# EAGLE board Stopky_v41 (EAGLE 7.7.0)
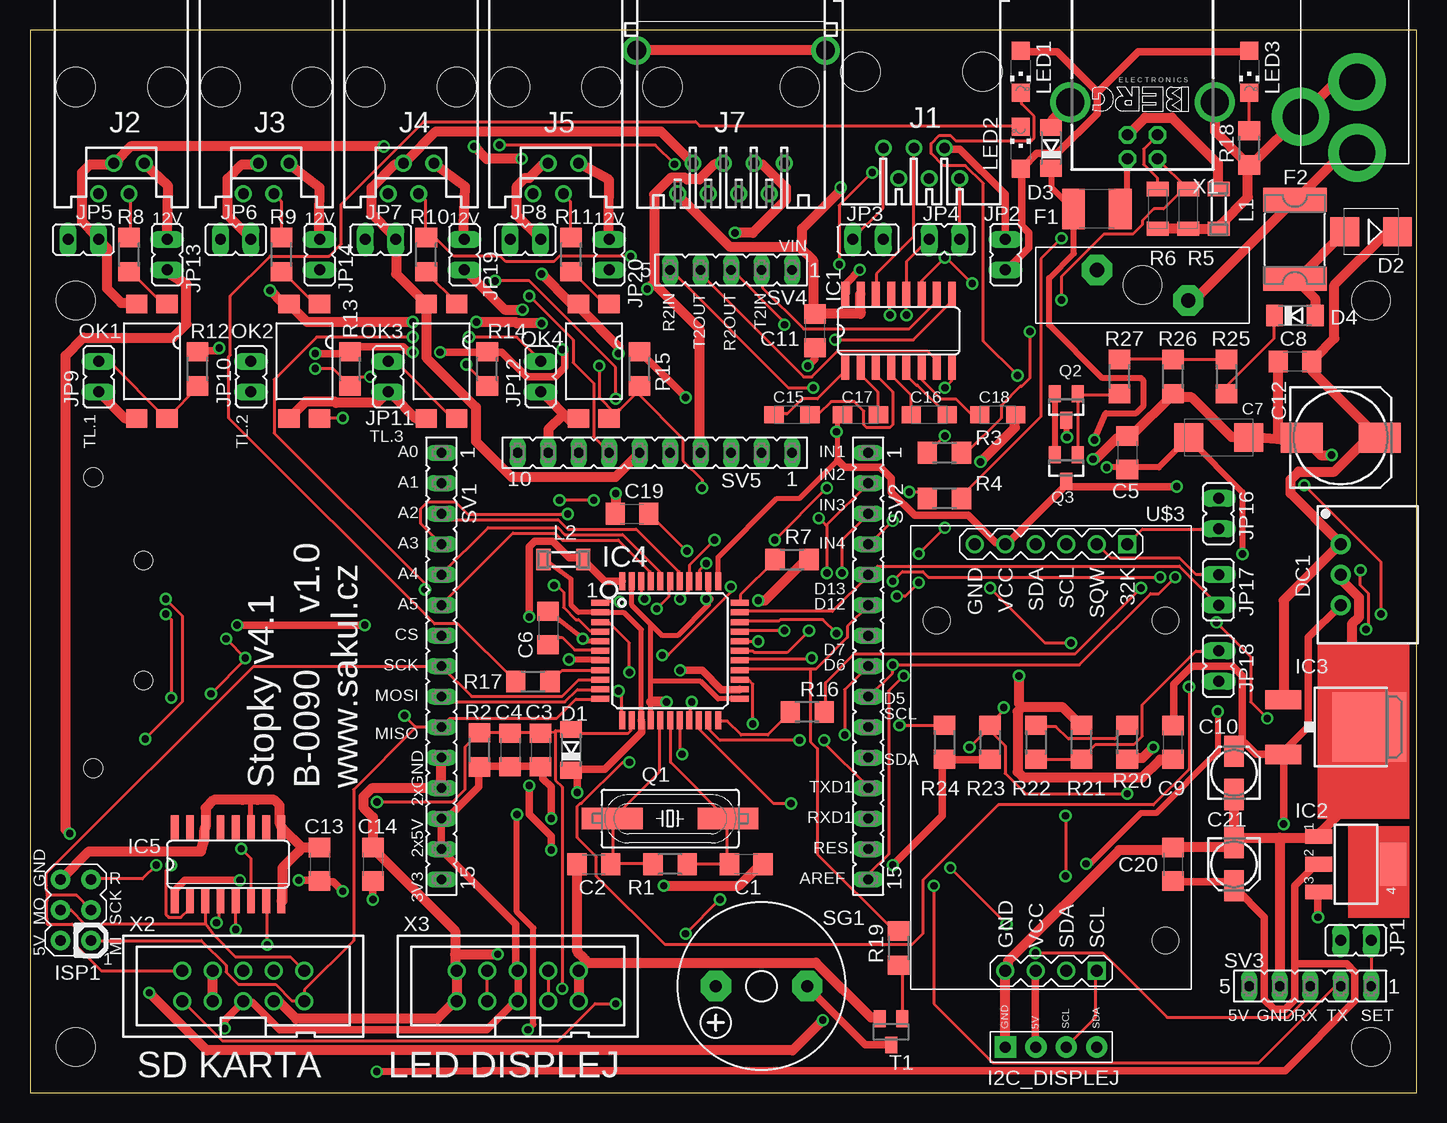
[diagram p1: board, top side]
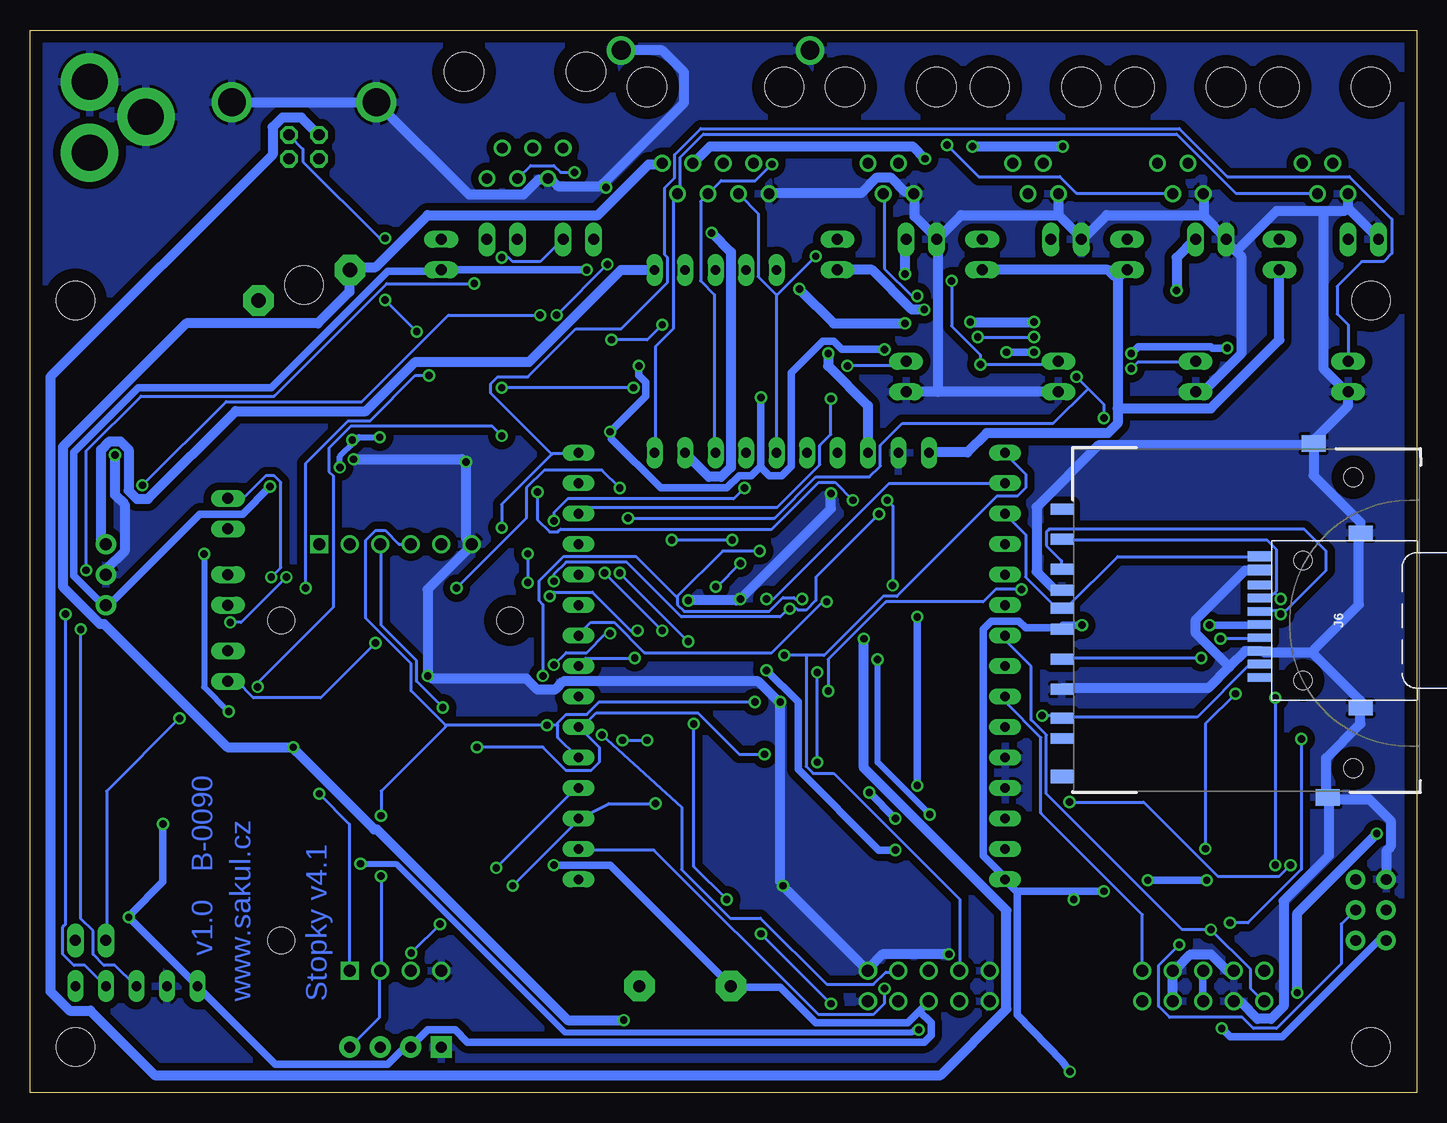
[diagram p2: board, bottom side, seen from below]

Size 115.55 x 88.57 mm. Coordinates in mm from the lower left corner, seen from the top.
Outline: 0,0 115.55,0 115.55,88.57 0,88.57 0,0
Copper layers (1*16): Top 0.035mm / dielectric 1.5mm / Bottom 0.035mm
Design rules "default": minimum track width 10mil, minimum drill 24mil, track to track 8mil, track to pad 8mil, pad to pad 8mil, via to via 8mil, smd to smd 8mil, copper to edge 40mil, drill to drill 8mil, minimum pad ring 10mil, minimum via ring 8mil, stop-mask expansion 4mil, vias tented up to drill 0mil, thermal gap 10mil
Net classes: 0 default: width 0.203 mm, drill 0.406 mm, clearance 0.203 mm; 1 12V: width 0.813 mm, drill 0.406 mm, clearance 0.203 mm; 2 5V: width 0.61 mm, drill 0.406 mm, clearance 0.203 mm; 3 GND: width 0.813 mm, drill 0.406 mm, clearance 0.203 mm; 4 3V3: width 0.61 mm, drill 0.406 mm, clearance 0.203 mm; 5 USB: width 0.508 mm, drill 0.406 mm, clearance 0.203 mm
Holes 3.2 mm at 3.81,3.81 111.76,3.81 3.81,66.04 111.76,66.04

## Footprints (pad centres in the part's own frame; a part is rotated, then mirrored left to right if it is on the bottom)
C1206 = smd 1.6 x 1.8: 1 -1.4,0; 2 1.4,0
SMC_C = smd 2.4 x 2.4: + -2.5,0; - 2.5,0
153CLV-0405 = smd 2.6 x 1.6: + 1.8,0; - -1.8,0
153CLV-0810 = smd 3.5 x 2.5: + 3.25,0; - -3.25,0
SMC_A = smd 1.6 x 1.4: + -1.5,0; - 1.5,0
SOD80C = smd 1.4 x 1.8: A 1.7,0; C -1.7,0
SMB = smd 2.4 x 2.4: A 2.2,0; C -2.2,0
SIP3 = drill 1 pad 1.676: 1 -2.54,0; 2 0,0; 3 2.54,0
L1812 = smd 1.9 x 3.4: 1 -1.95,0; 2 1.95,0
2920L = smd 2 x 5.3: 1 -3.3,0; 2 3.3,0
I2C_HEADER_FOOTPRINT = drill 0.9 pad 1.778: 5V -1.27,0; SCL 1.27,0; SDA 3.81,0 | drill 0.9 pad 1.778 square: GND -3.81,0
SO16 = smd 0.66 x 2.032: 1 -4.445,-3.073; 2 -3.175,-3.073; 3 -1.905,-3.073; 4 -0.635,-3.073; 5 0.635,-3.073; 6 1.905,-3.073; 7 3.175,-3.073; 8 4.445,-3.073; 9 4.445,3.073; 10 3.175,3.073; 11 1.905,3.073; 12 0.635,3.073; 13 -0.635,3.073; 14 -1.905,3.073; 15 -3.175,3.073; 16 -4.445,3.073
SOT223 = smd 1.219 x 2.235: 1 -2.311,-3.099; 2 0,-3.099; 3 2.311,-3.099 | smd 3.6 x 2.2: 4 0,3.099
DPACK = smd 1.6 x 3: 1 -2.28,-4.8; 3 2.28,-4.8 | smd 5.8 x 6.2: 4 0,2.38
TQFP44 = smd 1.5 x 0.5: 1 -5.8,4; 2 -5.8,3.2; 3 -5.8,2.4; 4 -5.8,1.6; 5 -5.8,0.8; 6 -5.8,0; 7 -5.8,-0.8; 8 -5.8,-1.6; 9 -5.8,-2.4; 10 -5.8,-3.2; 11 -5.8,-4; 23 5.8,-4; 24 5.8,-3.2; 25 5.8,-2.4; 26 5.8,-1.6; 27 5.8,-0.8; 28 5.8,0; 29 5.8,0.8; 30 5.8,1.6; 31 5.8,2.4; 32 5.8,3.2; 33 5.8,4 | smd 0.5 x 1.5: 12 -4,-5.8; 13 -3.2,-5.8; 14 -2.4,-5.8; 15 -1.6,-5.8; 16 -0.8,-5.8; 17 0,-5.8; 18 0.8,-5.8; 19 1.6,-5.8; 20 2.4,-5.8; 21 3.2,-5.8; 22 4,-5.8; 34 4,5.8; 35 3.2,5.8; 36 2.4,5.8; 37 1.6,5.8; 38 0.8,5.8; 39 0,5.8; 40 -0.8,5.8; 41 -1.6,5.8; 42 -2.4,5.8; 43 -3.2,5.8; 44 -4,5.8
AVRISP = drill 0.9 pad 1.626: 1 -1.27,2.54; 2 1.27,2.54; 3 -1.27,0; 4 1.27,0; 5 -1.27,-2.54; 6 1.27,-2.54
520250-3 = drill 0.889: 1 -3.175,8.89; 2 -1.905,6.35; 3 -0.635,8.89; 4 0.635,6.35; 5 1.905,8.89; 6 3.175,6.35 | hole 3.251: -5.08,0; 5.08,0
215875-3 = drill 0.889: 1 -1.905,6.35; 2 -0.635,8.89; 3 0.635,6.35; 4 1.905,8.89 | hole 3.251: -3.81,0; 3.81,0
ATTEND-112 = smd 0.85 x 2: CD 5.35,8.62; GND 4.2,8.62 | smd 0.7 x 2: CLK -1.45,8.62; CMD 0.75,8.62; DAT0 -3.65,8.62; DAT1 -4.75,8.62; DAT2 2.95,8.62; DAT3 1.85,8.62; VDD -0.35,8.62; VSS -2.55,8.62 | smd 1.2 x 2: S1 -7.3,0.22; S2 7.3,0.22 | hole 1.5: -5,5.02; 5,5.02
555153-1 = drill 0.889: 1 -4.445,6.35; 2 -3.175,8.89; 3 -1.905,6.35; 4 -0.635,8.89; 5 0.635,6.35; 6 1.905,8.89; 7 3.175,6.35; 8 4.445,8.89 | drill 1.575 pad 2.184: G1 -7.874,-3.048; G2 7.874,-3.048 | hole 3.251: -5.715,0; 5.715,0
JP1 = drill 0.914 long: 1 0,-1.27; 2 0,1.27
SM-1206 = smd 1.2 x 1.8: 1 -1.65,0; 2 1.65,0
CHIPLED_1206 = smd 1.5 x 1.5: A 0,-1.75; C 0,1.75
SMD4-7 = smd 1.78 x 1.55: 1 -1.27,-4.77; 2 1.27,-4.77; 3 1.27,4.77; 4 -1.27,4.77
SM49 = smd 5.08 x 1.778: 1 -4.826,0; 2 4.826,0
SOT23 = smd 1 x 1.4: 1 -0.95,-1.1; 2 0.95,-1.1; 3 0,1.1
R1206 = smd 1.6 x 1.803: 1 -1.422,0; 2 1.422,0
CT/CN1206 = smd 1.2 x 1.8: 1 -1.65,0; 2 1.65,0
F/CM12P = drill 1.016 pad 2.54 octagon: + 3.81,0; - -3.81,0
FE15 = drill 0.813 long: 1 -17.78,0; 2 -15.24,0; 3 -12.7,0; 4 -10.16,0; 5 -7.62,0; 6 -5.08,0; 7 -2.54,0; 8 0,0; 9 2.54,0; 10 5.08,0; 11 7.62,0; 12 10.16,0; 13 12.7,0; 14 15.24,0; 15 17.78,0
FE05-1 = drill 0.813 long: 1 -5.08,0; 2 -2.54,0; 3 0,0; 4 2.54,0; 5 5.08,0
FE10 = drill 0.813 long: 1 -11.43,0; 2 -8.89,0; 3 -6.35,0; 4 -3.81,0; 5 -1.27,0; 6 1.27,0; 7 3.81,0; 8 6.35,0; 9 8.89,0; 10 11.43,0
SDCARD-SOCKET = smd 1.8 x 0.9: 1 -1,6.77; 2 -1,4.27; 3 -1,2.52; 4 -1,-0.73; 5 -1,-3.23; 6 -1,-5.73; 7 -1,-8.15; 8 -1,-9.85; 9 -1,9.27; CD -1,1.02 | smd 2 x 1.4: SH@1 20,14.75; SH@2 21.15,-14.75 | smd 1.8 x 1.1: WP -1,-13 | hole 1.55: 23.3,11.94; 23.3,-12.32
SL-1538 = drill 1.2 pad 2.54 octagon: P$1 3.81,-1.27; P$2 -3.81,1.27 | hole 3.2: 0,0
PJ-102A = drill 3 pad 4.8: RING 0.1,-3.39; RING_SW -4.6,-6.29; TIP 0.1,-9.29
RTC-DS3231-AT24C32 = drill 1 square: J1.1 -17.78,6.35; J2.1 17.78,3.81 | drill 1: J1.2 -17.78,3.81; J1.3 -17.78,1.27; J1.4 -17.78,-1.27; J1.5 -17.78,-3.81; J1.6 -17.78,-6.35; J2.2 17.78,1.27; J2.3 17.78,-1.27; J2.4 17.78,-3.81 | hole 2.2: -11.43,-9.525; -11.43,9.525; 15.24,9.525
PN61729-S = drill 0.95 octagon: 1 1.25,4.71; 2 -1.25,4.71; 3 -1.25,2.71; 4 1.25,2.71 | drill 2.3 pad 2.9: S1 -6.02,0; S2 6.02,0
PAK100/2500-10 = drill 1 pad 1.422: 1 -5.08,-1.27; 2 -5.08,1.27; 3 -2.54,-1.27; 4 -2.54,1.27; 5 0,-1.27; 6 0,1.27; 7 2.54,-1.27; 8 2.54,1.27; 9 5.08,-1.27; 10 5.08,1.27

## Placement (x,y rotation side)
C1  22pF  [C1206]  59.69,19.05 180 top
C2  22pF  [C1206]  46.99,19.05 0 top
C3  100nF  [C1206]  42.55,28.57 270 top
C4  100nF  [C1206]  40.01,28.57 270 top
C5  100nF  [C1206]  91.44,53.34 270 top
C6  1uF  [C1206]  43.18,38.73 270 top
C7  10uF  [SMC_C]  99.06,54.61 0 top
C8  100nF  [C1206]  105.41,60.96 0 top
C9  100nF  [C1206]  95.25,29.21 90 top
C10  10uF/10V  [153CLV-0405]  100.33,26.67 90 top
C11  100nF  [C1206]  65.41,63.5 270 top
C12  220uF/35V  [153CLV-0810]  109.22,54.61 0 top
C13  100nF  [C1206]  24.13,19.05 270 top
C14  100nF  [C1206]  28.57,19.05 270 top
C15  1uF  [SMC_A]  63.5,56.52 0 top
C16  1uF  [SMC_A]  74.93,56.52 0 top
C17  1uF  [SMC_A]  69.22,56.52 180 top
C18  1uF  [SMC_A]  80.64,56.52 180 top
C19  100nF  [C1206]  50.16,48.26 0 top
C20  100nF  [C1206]  95.25,19.05 270 top
C21  10uF/10V  [153CLV-0405]  100.33,19.05 270 top
D1  1N4148  [SOD80C]  45.09,28.57 90 top
D2  STPS340U (TME)  [SMB]  111.76,71.75 180 top
D3  5V6  [SOD80C]  85.09,78.74 90 top
D4  1N4148  [SOD80C]  105.41,64.77 0 top
DC1  R-785.0-0.5  [SIP3]  109.22,43.18 270 top
F1  MF-MSMF050-2 500mA  [L1812]  88.9,73.66 180 top
F2  SL125-33 (TME)  [2920L]  105.41,71.12 90 top
I2C_DISPLEJ  I2C Display  [I2C_HEADER_FOOTPRINT]  85.09,3.81 0 top
IC1  MAX232  [SO16]  72.39,63.5 0 top
IC2  LM1117 3V3  [SOT223]  110.49,19.05 270 top
IC3  78M05 DPAK (LF50CDT)  [DPACK]  109.22,30.48 270 top
IC4  ATMEGA32U4-AU  [TQFP44]  53.34,36.83 0 top
IC5  4050D  [SO16]  16.51,19.05 0 top
ISP1  AVRISP-6  [AVRISP]  3.81,15.24 180 top
J1  [520250-3]  74.3,85.09 180 top
J2  [215875-3]  7.62,83.82 180 top
J3  [215875-3]  19.68,83.82 180 top
J4  [215875-3]  31.75,83.82 180 top
J5  [215875-3]  43.81,83.82 180 top
J6  ATTEND-MICROSD-112  [ATTEND-112]  4.45,39.37 90 bottom
J7  [555153-1]  58.42,83.82 180 top
JP1  [JP1]  110.49,12.7 270 top
JP2  [JP1]  81.28,69.85 0 top
JP3  [JP1]  69.85,71.12 90 top
JP4  [JP1]  76.2,71.12 270 top
JP5  [JP1]  4.45,71.12 90 top
JP6  [JP1]  17.14,71.12 90 top
JP7  [JP1]  29.21,71.12 90 top
JP8  [JP1]  41.27,71.12 90 top
JP9  [JP1]  5.71,59.69 0 top
JP10  [JP1]  18.41,59.69 0 top
JP11  [JP1]  29.84,59.69 0 top
JP12  [JP1]  42.55,59.69 0 top
JP13  [JP1]  11.43,69.85 0 top
JP14  [JP1]  24.13,69.85 0 top
JP16  [JP1]  99.06,48.26 180 top
JP17  [JP1]  99.06,41.91 180 top
JP18  [JP1]  99.06,35.56 180 top
JP19  [JP1]  36.2,69.85 0 top
JP20  [JP1]  48.26,69.85 0 top
L1  MH2029-300Y (1206)  [SM-1206]  99.06,73.66 90 top
L2  MH2029-300Y (1206)  [SM-1206]  44.45,44.45 180 top
LED1  [CHIPLED_1206]  82.55,85.09 180 top
LED2  [CHIPLED_1206]  82.55,78.74 0 top
LED3  [CHIPLED_1206]  101.6,85.09 180 top
OK1  SFH618A  [SMD4-7]  10.16,60.96 180 top
OK2  SFH618A  [SMD4-7]  22.86,60.96 180 top
OK3  SFH618A  [SMD4-7]  34.29,60.96 180 top
OK4  SFH618A  [SMD4-7]  46.99,60.96 180 top
Q1  16MHz  [SM49]  53.34,22.86 0 top
Q2  IRLML6402TRPBF  [SOT23]  86.36,57.15 180 top
Q3  IRLML6402TRPBF  [SOT23]  86.36,52.07 180 top
R1  1M  [R1206]  53.34,19.05 0 top
R2  10K  [R1206]  37.47,28.57 270 top
R3  22R  [R1206]  76.2,53.34 0 top
R4  22R  [R1206]  76.2,49.53 0 top
R5  B72520T040M62 (Varistor)  [CT/CN1206]  96.52,73.66 270 top
R6  B72520T040M62 (Varistor)  [CT/CN1206]  93.98,73.66 270 top
R7  10K  [R1206]  63.5,44.45 180 top
R8  3K9  [R1206]  8.26,69.85 270 top
R9  3K9  [R1206]  20.95,69.85 270 top
R10  3K9  [R1206]  33.02,69.85 270 top
R11  3K9  [R1206]  45.09,69.85 270 top
R12  10K  [R1206]  13.97,60.33 270 top
R13  10K  [R1206]  26.67,60.33 270 top
R14  10K  [R1206]  38.1,60.33 270 top
R15  10K  [R1206]  50.8,60.33 270 top
R16  1K  [R1206]  64.77,31.75 0 top
R17  1K  [R1206]  41.91,34.29 180 top
R18  1K  [R1206]  101.6,78.74 90 top
R19  10K  [R1206]  72.39,12.06 90 top
R20  10K  [R1206]  91.44,29.21 270 top
R21  2K2  [R1206]  87.63,29.21 270 top
R22  1K  [R1206]  83.82,29.21 90 top
R23  10K  [R1206]  80.01,29.21 90 top
R24  10K  [R1206]  76.2,29.21 90 top
R25  10K  [R1206]  99.69,59.69 90 top
R26  2K2  [R1206]  95.25,59.69 270 top
R27  10R  [R1206]  90.81,59.69 270 top
SG1  F/CM12P  [F/CM12P]  60.96,8.89 180 top
SV1  [FE15]  34.29,35.56 270 top
SV2  [FE15]  69.85,35.56 270 top
SV3  HC11/12  [FE05-1]  106.68,8.89 180 top
SV4  [FE05-1]  58.42,68.58 180 top
SV5  [FE10]  52.07,53.34 180 top
T1  BC846  [SOT23]  71.75,5.08 180 top
U1  [SDCARD-SOCKET]  28.57,39.37 0 bottom
U$1  ASL-1538 2A  [SL-1538]  92.71,67.31 180 top
U$2  2.1MMJACKTHM  [PJ-102A]  110.49,87.63 0 top
U$3  RTC-DS3231-AT24C32  [RTC-DS3231-AT24C32]  85.09,27.94 270 top
X1  PN61729-S  [PN61729-S]  92.71,82.55 180 top
X2  2510-  [PAK100/2500-10]  17.78,8.89 0 top
X3  2510-  [PAK100/2500-10]  40.64,8.89 0 top

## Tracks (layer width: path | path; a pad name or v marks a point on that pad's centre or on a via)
+3V3  (via drill 0.61)
  Top 0.61: C20.2 95.33,17.6 99.9,17.6 100.24,17.26 C21.+ 100.47,17.03 102.87,14.63 102.87,7.77 103.67,6.97 104.58,6.97 105.39,7.77 105.39,10.74 | 105.39,10.74 105.39,17.26 107.1,18.97 107.33,18.97 IC2.2 | v26.06,16.8 25.26,17.6 24.23,17.6 C13.2 23.89,17.72 v22.4,17.72 | v28.57,16.12 C14.2 | v27.89,38.98 v17.26,38.98 | v17.49,17.72 12.92,17.72 12.12,16.92 12.12,16 IC5.1 | 105.39,10.74 109.73,10.74 110.41,10.06 110.41,7.66 104.58,1.83 37.72,1.83 v28.89,1.76
  Bottom 0.61: 33.26,16.8 33.38,16.8 34.29,17.72 SV1.15 34.4,18.06 36.12,19.77 36.12,38.63 35.43,39.32 33.15,39.32 32.58,38.75 29.6,38.75 U1.4 29.49,38.98 v27.89,38.98 | 33.26,16.8 28.57,16.8 | 28.57,16.8 v26.06,16.8 | 28.57,16.8 v28.57,16.12 | v17.26,38.98 13.14,38.98 J6.VDD | v22.4,17.72 v17.49,17.72 | v28.89,1.76 29.53,2.63 33.26,6.51 33.26,16.8
+5V  (via drill 0.61)
  Top 0.406: IC4.14 50.94,38.59 49.53,40.01 47.56,40.01 IC4.2 45.7,40.03 45.09,40.64 45.09,42.8 L2.2 | IC4.34 57.34,44.64 62.23,49.53 64.14,49.53 67.31,52.7 67.31,55.09 67.31,56.11 C17.-
  Top 0.61: R23.1 80.01,27.77 76.24,27.77 R24.1 76.01,27.55 76.01,23.09 v71.89,18.97 | v16.23,5.37 16.23,6.06 17.72,7.54 X2.5 18.06,7.54 18.52,7.54 20.8,5.26 38.06,5.26 40.35,7.54 X3.5 40.69,7.66 40.69,10.06 X3.6 40.46,10.4 40.46,14.06 34.4,20.12 SV1.14 SV1.13 34.52,22.97 34.86,22.97 37.38,25.49 37.38,26.86 R2.2 37.49,27.2 40.01,27.2 C4.2 40.23,27.2 42.52,27.2 C3.2 42.75,26.98 42.75,26.18 43.43,25.49 v43.43,22.86 | IC4.14 50.98,30.86 50.98,30.06 47.89,26.98 45.15,26.98 D1.C 45.61,26.75 v45.61,25.03 | v15.77,62.06 15.54,61.84 14.06,61.84 R12.1 | v23.77,61.61 26.52,61.61 26.63,61.72 R13.1 26.98,61.84 27.32,62.18 31.09,62.18 31.55,61.72 v31.89,61.72 | v34.18,61.72 38.06,61.72 R14.1 38.41,61.72 39.32,61.72 41.38,59.66 43.78,59.66 44.58,60.47 44.58,61.72 v44.35,61.95 | v64.81,60.58 65.38,61.15 65.38,62.06 C11.2 | v67.21,55.09 67.31,55.09 | v54.63,57.95 50.86,61.72 R15.1 | 67.31,52.7 67.89,52.12 70.87,52.12 71.78,51.21 71.78,50.06 73.72,48.12 78.18,48.12 80.47,45.83 81.04,45.83 U$3.J1.5 81.38,45.72 86.3,50.63 86.3,50.86 Q3.3 86.53,50.52 v95.56,50.52 | JP2.1 81.38,68.58 83.21,70.41 83.21,71.67 82.64,72.24 82.64,76.92 LED2.A 82.75,77.15 83.9,78.3 85.61,78.3 88.92,81.61 88.92,83.44 | 88.92,83.44 85.61,86.75 82.64,86.75 LED1.A | LED3.A 101.5,86.75 92.35,86.75 89.15,83.55 88.92,83.44 | v69.15,68.58 68.01,67.44 68.01,66.64 IC1.16 | 101.04,29.26 101.04,34.75 100.24,35.55 96.81,35.55 95.33,34.06 95.33,30.63 C9.2 | 101.04,29.26 100.36,28.57 C10.+ | IC3.3 104.36,28.23 102.18,28.23 101.27,29.15 101.04,29.26 | DC1.3 106.53,37.95 106.53,30.52 104.47,28.46 IC3.3
  Top 0.61: U$3.J2.3 83.78,10.06 83.78,3.89 I2C_DISPLEJ.5V | v107.33,14.63 107.33,16.69 IC2.3 | v104.47,22.4 104.47,27.89 IC3.3
  Bottom 0.61: v71.89,18.97 67.21,18.97 57.15,8.91 SG1.+ 56.92,8.8 53.03,8.8 50.06,5.83 42.41,5.83 41.43,6.8 | X2.5 17.83,7.66 17.83,10.06 X2.6 | v16.23,5.37 15.54,4.69 11.2,4.69 3.2,12.69 2.63,12.69 ISP1.2 | v43.43,22.86 v45.61,25.03 | 41.43,6.8 40.69,7.54 X3.5 | v15.77,62.06 17.03,62.06 17.14,62.18 23.2,62.18 v23.77,61.61 | v31.89,61.72 v34.18,61.72 | v64.81,60.58 64.81,59.78 64.24,59.21 64.24,58.06 v67.21,55.09 67.09,54.86 67.09,54.52 62.98,50.41 57.49,50.41 56.46,51.44 55.44,51.44 54.63,52.23 | 54.63,52.23 v54.63,57.95 | v44.35,61.95 47.89,61.95 48.58,62.64 49.49,62.64 52.12,60.01 52.12,52.23 52.92,51.44 53.95,51.44 54.52,52.01 54.63,52.23 | v69.15,68.58 JP2.1 81.5,68.47 85.72,68.47 95.44,58.75 106.53,58.75 111.9,53.38 111.9,43.09 109.5,40.69 109.27,40.69 DC1.3 108.93,40.69 101.38,48.23 97.84,48.23 v95.56,50.52 | v104.47,22.4 104.47,17.6 107.21,14.86 v107.33,14.63 101.61,8.91 SV3.5 101.38,8.69 95.1,2.4 85.72,2.4 84.35,3.77 83.9,3.77 I2C_DISPLEJ.5V 83.67,4 82.41,5.26 80.12,5.26 79.1,4.23 41.03,4.23 40.46,4.8 40.46,5.83 41.43,6.8
+12V  (via drill 0.61)
  Top 0.813: v41.03,65.27 39.55,65.27 36.23,68.58 JP19.1 | v93.61,28.8 92.7,27.89 91.44,27.89 R20.2 | JP13.1 11.43,68.35 13.03,67.39 13.03,64.06 11.9,62.93 4.46,62.93 2.97,61.44 2.97,21.95 v3.31,21.6 | v9.94,8.34 14.74,3.54 63.55,3.54 v66.06,6.06
  Bottom 0.813: 24.92,57.04 24.92,67.89 24.23,68.58 JP14.1 25.26,68.12 25.72,68.58 JP19.1 | 24.92,57.04 24.92,55.78 25.72,54.98 35.84,54.98 37.44,53.38 40.58,53.38 SV5.10 | JP13.1 11.43,62.75 17.14,57.04 24.92,57.04 | JP20.1 45.38,68.58 42.06,65.27 v41.03,65.27 | J7.1 62.87,77.38 64.01,77.38 68.24,73.15 82.41,73.15 86.75,68.81 88.58,68.81 U$1.P$1 88.92,68.58 88.92,66.75 91.55,64.12 102.53,64.12 112.81,53.84 112.81,42.18 109.73,39.09 109.39,39.09 99.1,28.8 v93.61,28.8 93.38,28.46 86.87,21.95 86.64,21.95 70.75,6.06 v66.06,6.06 | v3.31,21.6 9.94,14.97 v9.94,8.34
A0  (via drill 0.61)
  Top 0.254: X3.3 38.06,7.66 38.06,10.06 X3.4 | v56.35,44.12 55.78,43.55 55.78,42.63 IC4.36 | v58.41,42.18 58.41,41.72 53.15,36.46 v52.69,36.46
  Bottom 0.254: v56.35,44.12 58.29,42.18 v58.41,42.18 | 50.86,36.46 49.38,36.46 44.46,41.38 43.32,41.38 34.98,49.72 33.26,49.72 32.58,50.41 32.58,51.55 34.29,53.26 SV1.1 | 50.86,36.46 v52.69,36.46 | 50.86,36.46 50.86,27.2 50.29,26.63 48.58,26.63 38.06,16.12 38.06,10.17 X3.4
A1  (via drill 0.61)
  Top 0.254: v54.18,41.15 54.86,41.83 54.86,42.52 IC4.37 54.98,42.75 54.98,44.01 v57.04,46.06 | v86.75,37.49 84.58,37.49 v80.01,42.06 | v62.06,46.06 v66.41,50.41
  Bottom 0.254: v54.18,41.15 53.61,41.15 44.01,50.75 34.29,50.75 SV1.2 | JP18.2 98.3,34.29 96.93,32.92 91.33,32.92 v86.75,37.49 | v80.01,42.06 74.18,47.89 74.18,50.41 72.69,51.89 67.89,51.89 v66.41,50.41 | v57.04,46.06 v62.06,46.06
A2
  Top 0.254: IC4.38 54.06,42.63 54.06,43.43 50.52,46.98 44.81,46.98 44.01,47.78 34.75,47.78 34.29,48.23 SV1.3
  Bottom 0.254: SV1.3 34.29,48.23 32.58,46.52 32.58,42.98 30.06,40.46 29.6,40.46 U1.CD 29.49,40.46 29.15,40.46 24.92,44.69 13.14,44.69 J6.CD
A3  (via drill 0.61)
  Top 0.254: v52.23,40.35 53.26,41.38 53.26,42.52 IC4.39 | v44.81,48.23 36.46,48.23 35.43,49.26 33.15,49.26 32.58,48.69 32.58,47.43 SV1.4 | v103.1,31.2 101.73,32.58 101.73,36.35 v98.87,39.2 | v94.18,42.98 74.87,42.98 74.41,43.43 72.69,43.43 v71.89,42.63
  Bottom 0.254: v44.81,48.23 50.06,42.98 50.06,41.03 50.86,40.23 51.55,40.23 51.66,40.35 v52.23,40.35 52.35,40.35 53.03,39.66 61.27,39.66 65.84,44.23 70.87,44.23 71.89,43.2 v71.89,42.63 | v103.1,31.2 109.16,25.15 109.16,12.8 JP1.1 | v98.87,39.2 97.95,39.2 v94.18,42.98
A4
  Top 0.254: IC4.40 52.46,42.63 52.46,43.43 49.38,46.52 44.58,46.52 44.01,47.09 38.18,47.09 34.29,43.2 SV1.5
A5
  Top 0.254: IC4.41 51.66,42.63 51.66,43.43 49.03,46.06 44.35,46.06 43.78,46.63 40.23,46.63 34.29,40.69 SV1.6
AREF  (via drill 0.61)
  Top 0.254: v51.21,41.15 50.98,41.38 50.98,42.52 IC4.42 | v54.75,45.15 51.66,48.23 C19.2 | v72.81,34.75 71.55,33.49 71.55,19.89 69.95,18.29 69.95,17.83 SV2.15
  Bottom 0.254: v51.21,41.15 51.78,41.15 51.89,41.26 52.81,41.26 53.95,40.12 61.04,40.12 61.61,40.69 61.61,41.38 | 61.61,41.38 57.84,45.15 v54.75,45.15 | v72.81,34.75 72.81,40.69 73.15,41.03 73.15,42.63 71.09,44.69 65.04,44.69 61.72,41.38 61.61,41.38
CS  (via drill 0.61)
  Top 0.254: v60.24,30.75 60.24,34.06 59.89,34.4 59.21,34.4 IC4.25 | v54.63,13.26 v57.49,16.12 | v48.81,7.43 47.09,7.43 44.01,4.34 16,4.34 12.8,7.54 X2.1 | v17.14,13.6 IC5.5
  Bottom 0.254: v60.24,30.75 60.24,18.86 v57.49,16.12 | v48.81,7.43 v54.63,13.26 | X2.1 12.8,7.66 13.83,8.69 13.83,10.29 v17.14,13.6 19.55,13.6 30.86,24.92 30.86,29.83 32.12,31.09 32.12,35.55 34.29,37.72 SV1.7
D5  (via drill 0.61)
  Top 0.254: v67.21,38.29 66.06,39.43 62.52,39.43 62.41,39.32 59.21,39.32 IC4.31 | SV2.9 69.95,33.03 71.89,34.98 v71.89,35.66 87.44,35.66 93.38,41.6 94.07,41.6 v95.44,42.98
  Bottom 0.254: v67.21,38.29 67.55,38.29 69.15,36.69 70.87,36.69 v71.89,35.66 | v95.44,42.98 94.64,43.78 94.64,50.86 95.21,51.44 95.9,51.44 97.73,49.61 98.98,49.61 JP16.1
D6  (via drill 0.61)
  Top 0.254: X3.7 43.2,7.66 43.2,10.06 X3.8 | v65.15,36.23 65.04,36.12 59.21,36.12 IC4.27 | v67.89,29.83 67.89,33.6 SV2.8
  Bottom 0.254: v65.15,36.23 69.27,36.23 69.84,35.66 SV2.8 | v67.89,29.83 61.24,23.81 61.24,18.61 57.2,14.57 54.69,14.57 49.15,9.03 45.26,9.03 44.23,10.06 43.2,10.06 X3.8
D7  (via drill 0.61)
  Top 0.254: v49.15,40.92 47.55,40.92 IC4.1
  Bottom 0.254: v49.15,40.92 49.49,40.92 53.72,36.69 64.35,36.69 66.86,39.2 68.81,39.2 69.84,38.18 SV2.7
D12
  Top 0.254: 65.04,35.32 65.49,35.32 68.12,37.95 68.12,38.86 69.84,40.58 SV2.6 | 65.04,35.32 59.21,35.32 IC4.26 | 65.04,35.32 65.04,29.26 65.61,28.69 65.61,19.89 72.01,13.49 72.35,13.49 R19.2
D13
  Top 0.254: IC4.32 59.21,40.12 66.86,40.12 69.84,43.09 SV2.5 69.95,43.2 70.64,43.89 95.78,43.89 98.98,40.69 JP17.2
GND  (via drill 0.61)
  Top 0.406: IC4.35 56.54,41.15 56.54,40.66 53.98,38.1 52.7,38.1 51.74,39.06 | 51.74,39.06 50.16,40.64 50.16,42.6 IC4.43 | IC4.23 57.34,32.83 55.88,34.29 51.74,34.29 | IC4.15 51.74,32.58 51.74,34.29 | 51.74,34.29 51.74,39.06 | 18.34,24.42 18.34,22.19 IC5.11
  Top 0.813: DC1.2 109.27,43.09 109.27,42.75 110.76,41.26 110.76,39.65 110.19,39.08 110.19,31.89 111.56,30.52 IC3.4 111.33,30.18 111.33,25.49 107.56,21.72 IC2.1 107.33,21.26 104.13,21.26 | I2C_DISPLEJ.GND 81.27,3.89 81.27,10.06 U$3.J2.4 81.5,10.52 81.5,10.97 90.75,20.23 94.87,20.23 C20.1 95.33,20.46 99.9,20.46 100.24,20.8 C21.- | 104.13,21.26 100.7,21.26 100.58,21.14 C21.- | C10.- 100.36,24.8 100.36,21.49 C21.- | 104.13,21.26 104.13,8.91 SV3.4 | 82.64,32.12 82.3,31.77 82.3,26.75 82.75,26.29 92.7,26.29 94.18,27.77 95.21,27.77 C9.1 | 82.64,32.12 86.07,32.12 87.55,30.63 R21.1 | v79.21,52.58 82.07,55.44 82.07,56.46 C18.+ | 104.01,54.67 104.01,60.92 C8.1 | 104.01,54.67 105.96,54.63 C12.- 106.3,54.41 107.56,53.15 v108.47,53.15 | 104.01,54.67 104.31,54.45 101.96,54.63 101.61,54.63 C7.- 101.16,54.63 100.13,54.63 96.81,57.95 95.56,57.95 R26.2 95.21,58.18 91.78,54.75 C5.1 91.1,54.52 90.53,54.52 88.81,52.81 v88.58,52.81 | v82.41,34.75 82.41,32.46 82.64,32.12 | v48.81,49.95 48.81,48.35 C19.1 | v56.35,41.15 56.54,41.15 | v60.69,41.03 61.27,41.03 64.58,44.35 64.81,44.35 R7.1 | 46.41,10.86 65.49,10.86 70.07,6.29 70.75,6.29 T1.2 | 46.41,10.86 45.72,10.17 X3.10 X3.9 | C2.1 45.61,18.97 45.61,11.77 46.18,11.2 46.41,10.86 | v52.81,17.26 59.09,17.26 60.81,18.97 61.04,18.97 C1.1 | v53.03,32.58 51.74,32.58 | X2.3 15.2,7.66 15.2,10.06 X2.4 | SV1.11 SV1.12 34.29,25.38 28.46,25.38 27.77,24.69 27.77,23.77 28.57,22.97 C14.1 28.8,20.12 35.43,13.49 35.43,11.54 | 35.43,11.54 35.43,10.52 X3.2 35.55,10.06 35.55,7.66 X3.1 35.2,7.43 33.95,6.17 22.17,6.17 20.8,7.54 20.34,7.54 X2.7 | OK1.3 8.8,56.24 7.89,56.24 5.71,58.41 JP9.1
  Top 0.813: 22.63,20.46 24.12,20.46 C13.1 | 22.63,20.46 21.03,22.06 IC5.9 20.8,22.52 20.8,23.95 20.34,24.41 18.97,24.41 18.34,24.42 17.72,24.41 15.32,24.41 14.63,23.72 14.63,22.17 IC5.14 14.52,21.72 14.52,21.03 14.24,20.12 4.92,20.12 2.63,17.83 ISP1.6 | IC5.8 21.03,16 21.03,18.75 22.4,20.12 22.63,20.46 | R6.2 94.07,72.01 96.47,72.01 R5.2 96.93,72.01 98.98,72.01 L1.1 99.21,72.35 101.5,74.64 101.5,77.27 R18.1 | R18.1 101.96,77.5 105.84,81.38 U$2.RING_SW 106.19,81.61 108.81,84.24 110.53,84.24 U$2.RING | X1.S1 98.75,82.53 98.75,80.12 101.27,77.61 R18.1 | J7.G1 J7.G2 | D3.A 85.15,80.47 85.15,81.04 86.64,82.53 X1.S2 | SV5.9 43.2,55.28 44.45,56.53 OK4.3 45.15,55.89 42.63,58.41 JP12.1 | OK2.3 21.6,56.24 22.97,57.61 25.38,57.61 25.49,57.49 28.92,57.49 JP11.1 30.18,58.18 32.12,56.24 32.92,56.24 OK3.3 | IC1.15 69.15,66.52 69.15,65.49 69.22,64.92 65.49,64.92 C11.1 65.27,65.27 65.27,69.38 64.12,70.52 | 64.12,70.52 58.29,70.52 53.95,74.87 J7.8 | v67.55,75.44 67.55,75.21 64.35,72.01 64.35,70.87 64.12,70.52 | 35.43,11.54 v38.98,11.54
  Bottom 0.813: v88.58,52.81 79.55,52.81 v79.21,52.58 79.21,46.18 78.75,45.72 U$3.J1.6 78.98,45.38 82.41,41.95 v82.41,34.75 82.07,34.52 74.18,34.52 73.27,33.6 71.78,33.6 71.09,34.29 54.86,34.29 53.38,32.8 v53.03,32.58 53.03,17.6 v52.81,17.26 45.72,10.17 X3.10 45.38,10.4 45.67,10.4 44.53,11.54 v38.98,11.54 | v48.81,49.95 48.81,48.69 v56.35,41.15 56.69,41.03 v60.69,41.03 | v108.47,53.15 108.47,49.84 107.67,49.03 107.67,45.15 109.16,43.66 109.16,43.2 DC1.2 | X2.7 20.34,7.66 20.34,10.06 X2.8 20,10.4 18.86,11.54 17.14,11.54 15.77,10.17 15.32,10.17 X2.4 | U1.3 29.6,41.95 30.18,41.95 31.66,43.43 31.66,48.81 26.52,53.95 8.8,53.95 8.69,54.06 U1.SH@1 | U1.SH@1 8.57,53.61 8.57,51.44 4.69,47.55 4.69,46.75 J6.S2 4.8,46.29 4.8,40.69 8.46,37.03 8.69,36.69 | U1.SH@1 8.46,54.52 5.71,57.26 JP9.1 6.06,58.64 7.77,60.35 7.77,73.5 | 15.6,35.49 14.29,36.8 13.14,36.8 J6.VSS 12.69,36.69 8.69,36.69 | 15.6,35.49 17.37,33.72 29.49,33.72 U1.6 | 15.6,35.49 18.4,38.29 18.4,39.43 14.29,43.55 13.14,43.55 J6.GND | U1.SH@2 7.43,24.69 7.54,24.8 7.54,27.89 4.69,30.75 4.69,32 J6.S1 4.69,32.46 4.69,32.69 8.69,36.69 | ISP1.6 2.52,17.83 2.52,20.17 2.17,20.51 2.17,22.7 3.94,24.46 7.09,24.46 U1.SH@2 | X2.3 15.2,7.54 14.63,7.54 13.26,6.17 12.12,6.17 11.09,7.2 11.09,16 7.32,19.77 7.32,24.12 U1.SH@2 | J7.G1 62.87,86.87 61.04,85.04 61.04,82.53 67.84,75.72 | 67.84,75.72 68.01,75.55 71.55,75.55 72.01,76.01 J1.5 72.47,76.12 73.15,76.12 74.41,74.87 78.98,74.87 86.64,82.53 X1.S2 87.1,82.53 98.64,82.53 X1.S1 | 5.71,73.72 J2.4 | 5.71,73.72 3.2,71.21 JP5.2 | 17.72,73.15 17.72,73.04 15.89,71.21 JP6.2 15.66,70.75 15.03,70.12
  Bottom 0.813: 17.72,73.15 17.72,74.87 J3.4 | 15.03,70.12 14.63,69.72 14.63,61.61 17.72,58.52 18.4,58.52 JP10.1 | 7.77,73.5 11.66,73.5 15.03,70.12 | 7.77,73.5 6.06,73.5 5.71,73.72 | 39.89,58.41 29.95,58.41 JP11.1 | 39.89,58.41 42.52,58.41 JP12.1 | 29.83,73.15 29.83,74.87 J4.4 | 29.83,73.15 27.89,71.21 JP7.2 27.55,71.44 25.83,73.15 17.72,73.15 | JP8.2 40.01,71.21 41.83,73.04 41.83,74.87 J5.4 42.29,75.09 42.63,75.09 43.78,76.24 45.03,76.24 46.29,74.98 53.95,74.98 J7.8 | 29.83,73.15 37.95,73.15 39.66,71.44 JP8.2 | 39.89,58.41 39.89,70.75 JP8.2 | v67.55,75.44 67.84,75.72
  pour Bottom (isolate 0.61): 0.64,0.64 114.94,0.64 114.94,88.27 0,88.27 0,87.63 0.64,87.63
IN1  (via drill 0.61)
  Top 0.254: R12.2 14.06,58.86 11.43,56.24 OK1.4 11.32,56.24 6.63,60.92 5.71,60.92 JP9.2 | v64.92,38.52 63.09,36.69 60.35,36.69 60.24,36.8 59.21,36.8 IC4.28 | v72.24,41.38 72.92,41.38 v74.07,42.52 | v76.24,47.09 v74.07,44.92
  Bottom 0.254: v64.92,38.52 65.49,38.52 68.69,41.72 71.89,41.72 v72.24,41.38 | v74.07,44.92 v74.07,42.52 | v76.24,47.09 76.24,49.03 72.07,53.21 | 72.07,53.21 72.01,53.26 69.95,53.26 SV2.1 | JP9.2 5.71,64.01 6.63,64.92 6.63,67.21 4.57,69.27 2.74,69.27 2.06,69.95 2.06,72.81 5.6,76.35 15.77,76.35 19.77,80.35 59.66,80.35 61.84,78.18 61.84,76.24 62.64,75.44 62.64,69.84 62.41,69.61 62.41,67.55 66.29,63.66 70.07,63.66 74.07,59.66 76.58,59.66 77.15,59.09 77.15,58.29 72.07,53.21
IN2  (via drill 0.61)
  Top 0.254: v26.06,56.24 24.23,56.24 OK2.4 | v28.35,59.66 27.43,59.66 26.75,58.98 R13.2 26.63,58.98 25.26,60.35 v23.77,60.35 | v60.69,37.6 59.21,37.6 IC4.29 | 66.41,47.32 v66.41,43.32 | 66.41,47.32 69.84,50.75 SV2.2 | v65.72,47.89 66.29,47.32 66.41,47.32
  Bottom 0.254: v26.06,56.24 26.06,57.38 27.38,58.69 | v28.35,59.66 27.38,58.69 | v23.77,60.35 23.2,60.92 18.52,60.92 JP10.2 | v66.41,43.32 v60.69,37.6 | 27.38,58.69 30.29,55.78 42.86,55.78 44.69,53.95 44.69,52.23 45.61,51.32 50.06,51.32 53.49,47.89 v65.72,47.89
IN3  (via drill 0.61)
  Top 0.254: OK3.4 35.55,56.24 35.2,56.24 30.52,60.92 29.95,60.92 JP11.2 | v36.35,60.69 38.06,58.98 R14.2 | v62.87,38.52 59.21,38.52 IC4.30 | v67.67,43.32 67.67,46.06 69.84,48.23 SV2.3 | v38.75,67.67 41.6,67.67 48.81,60.47 v48.81,57.84
  Bottom 0.254: JP11.2 29.95,60.92 30.18,60.69 v36.35,60.69 36.35,61.49 38.75,63.89 v38.75,67.67 | v67.67,43.32 v62.87,38.52 | v48.81,57.84 48.81,54.86 49.72,53.95 49.72,52.35 53.26,48.81 69.38,48.81 69.84,48.35 SV2.3
IN4  (via drill 0.61)
  Top 0.254: v71.89,47.66 69.95,45.72 SV2.4 | v56.01,50.41 56.01,51.09 54.41,52.69 54.41,54.52 50.63,58.29 R15.2 50.75,58.86 50.75,58.52 49.15,56.92 49.03,56.92 48.35,56.24 OK4.4 48.69,56.69 47.43,57.95 v47.43,60.58 | v49.03,33.49 49.26,33.26 49.26,31.09 IC4.12 | v32.92,41.95 32.92,42.41 20.34,54.98 20.34,59.44 23.89,62.98 v31.89,62.98 | v36.58,62.98 40.58,62.98 42.52,61.04 JP12.2
  Bottom 0.254: v71.89,47.66 71.89,48.35 70.75,49.49 56.92,49.49 v56.01,50.41 | v49.03,33.49 49.03,36.12 44.23,40.92 36.12,40.92 35.09,41.95 v32.92,41.95 | v36.58,62.98 v31.89,62.98 | v47.43,60.58 42.98,60.58 42.63,60.92 JP12.2
J2-2
  Top 0.254: R8.1 8.34,71.32 8.34,74.87 J2.2
  Bottom 0.254: SV5.1 63.44,53.38 63.44,62.18 61.95,63.66 61.95,74.52 61.61,74.87 J7.2 61.49,74.98 61.38,75.09 61.38,77.95 59.44,79.9 20,79.9 15.09,74.98 8.34,74.98 J2.2
J2-3  (via drill 0.61)
  Top 0.813: OK1.2 8.8,65.84 7.59,65.84 6.4,67.03 6.4,70.41 5.71,71.09 JP5.1 5.49,71.44 4.34,72.58 4.34,76.71 5.02,77.38 6.97,77.38 J2.3 7.32,77.61 7.14,77.61 8.39,78.87 v29.49,78.87 | v58.75,71.67 60.24,71.67 62.98,74.41 62.98,75.44 61.04,77.38 60.35,77.38 J7.3 | v37.01,78.87 38.04,77.84 v40.97,77.84
  Bottom 0.813: v58.75,71.67 57.15,70.07 57.15,52.12 57.95,51.32 58.98,51.32 60.92,53.26 SV5.2 | v37.01,78.87 v29.49,78.87 | v40.97,77.84 42,78.87 58.86,78.87 60.24,77.5 J7.3
J3-2  (via drill 0.61)
  Top 0.254: R9.1 20.92,71.32 20.92,74.3 20.34,74.87 J3.2 | v39.13,78.98 52.12,78.98 v53.72,77.38
  Bottom 0.254: SV5.3 58.52,53.38 58.52,66.52 59.66,67.67 59.66,74.3 59.09,74.87 J7.4 58.98,74.98 57.95,76.01 55.09,76.01 v53.72,77.38 | v39.13,78.98 36.5,76.35 29.72,76.35 28.35,74.98 20.34,74.98 J3.2
J3-3  (via drill 0.61)
  Top 0.813: v20,66.86 21.03,65.84 21.49,65.84 OK2.2 21.83,65.49 23.09,64.24 v31.89,64.24 | J3.3 18.97,77.38 17.65,77.38 16.46,76.19 16.46,73.15 18.4,71.21 JP6.1 | 52.01,67.44 55.78,63.66 55.78,53.38 SV5.4 | 52.01,67.44 52.01,74.87 53.38,76.24 54.63,76.24 54.75,76.12 55.78,76.12 57.04,77.38 57.72,77.38 J7.5 | v37.2,64.24 40.46,64.24 40.58,64.12 v42.63,64.12 | v51.44,66.98 51.66,67.21 52.01,67.44
  Bottom 0.813: v20,66.86 20,69.61 18.52,71.09 JP6.1 | v37.2,64.24 v31.89,64.24 | v42.63,64.12 48.58,64.12 v51.44,66.98
J4-2  (via drill 0.61)
  Top 0.254: J4.2 32.46,74.87 32.92,74.41 32.92,71.32 R10.1 33.03,71.21 33.83,71.21 35.32,69.72 39.2,69.72 39.66,69.27 43.66,69.27 44.12,69.72 v50.06,69.72
  Bottom 0.254: 53.38,66.52 53.38,53.38 SV5.5 | 53.38,66.52 54.86,68.01 54.86,73.27 56.46,74.87 J7.6 | v50.06,69.72 53.26,66.52 53.38,66.52
J4-3
  Top 0.813: SV5.6 50.75,53.26 48.81,51.32 40.12,51.32 37.15,54.29 37.15,57.15 33.03,61.27 33.03,65.38 OK3.2 32.92,65.84 30.52,68.24 30.52,71.09 JP7.1 30.29,71.44 28.46,73.27 28.46,75.44 30.4,77.38 31.09,77.38 J4.3 31.43,77.72 33.83,80.12 52.58,80.12 55.21,77.5 J7.7
J5-2  (via drill 0.61)
  Top 0.254: R11.1 45.03,71.32 45.03,74.3 44.46,74.87 J5.2 | v41.6,66.41 45.26,62.75 45.26,60.86 46.98,59.14 46.98,54.69 48.23,53.43 48.23,53.38 SV5.7
  Bottom 0.254: v41.6,66.41 42.06,66.41 44.35,68.69 44.35,74.87 J5.2
J5-3  (via drill 0.61)
  Top 0.813: v42.63,68.24 45.03,65.84 45.72,65.84 OK4.2 45.83,65.38 49.03,62.18 v49.03,61.61 | J5.3 43.09,77.38 42.75,77.38 41.6,76.24 41.26,76.24 40.58,75.55 40.58,73.15 42.52,71.21 JP8.1
  Bottom 0.813: v42.63,68.24 42.63,71.09 JP8.1 | SV5.8 45.72,57.26 49.03,60.58 v49.03,61.61
MISO  (via drill 0.61)
  Top 0.254: ISP1.1 5.14,12.69 14.29,12.69 16.34,10.63 16.34,10.06 17.37,9.03 20.46,9.03 21.83,7.66 22.86,7.66 X2.9 22.86,8.57 26.98,12.69 26.98,25.26 32.12,30.4 32.12,30.52 | IC4.11 47.43,32.8 45.49,32.8 43.89,31.2 34.98,31.2 34.29,30.52 SV1.10 34.18,30.52 32.12,30.52 | v31.2,31.43 32.12,30.52
  Bottom 0.254: J6.DAT0 13.14,35.66 13.95,35.66 18.29,31.32 29.49,31.32 U1.7 29.49,31.43 v31.2,31.43
MOSI
  Top 0.254: IC4.10 47.43,33.6 45.61,33.6 44.58,32.58 34.63,32.58 34.29,32.92 SV1.9 | 14.63,14.06 15.27,13.2 17.14,11.32 21.72,11.32 22.86,10.17 X2.10 | 14.63,14.06 14.63,15.89 IC5.3 | 14.63,14.06 4.57,14.06 3.43,15.2 2.63,15.2 ISP1.4
  Bottom 0.254: SV1.9 34.29,32.58 31.32,29.6 31.32,23.32 22.86,14.86 X2.10
N$1  (via drill 0.61)
  Top 0.406: IC4.5 46.32,37.63 46.09,37.86 C6.1
  Top 0.813: L1.2 98.98,75.32 98.98,77.44 95.16,81.27 92.93,81.27 91.55,79.9 X1.4 | v46.06,37.83 46.09,37.86
  Bottom 0.813: v46.06,37.83 46.06,27.09 34.18,15.2 34.18,6.97 39.66,1.49 105.16,1.49 110.53,6.86 112.24,6.86 113.84,8.46 113.84,59.66 95.33,78.18 95.33,80.47 94.53,81.27 92.93,81.27 91.55,79.9 X1.4
N$2
  Top 0.508: X1.1 91.44,77.84 91.44,74.3 90.87,73.72 F1.1
N$3
  Top 0.254: R1.1 51.89,19.09 48.46,19.09 C2.2 48.58,19.2 48.58,22.75 Q1.1 48.58,22.86 52.46,26.75 52.46,30.98 IC4.16
N$4
  Top 0.254: R1.2 54.86,19.09 58.18,19.09 C1.2 58.06,19.2 58.06,22.75 Q1.2 58.06,22.86 53.38,27.55 53.38,30.98 IC4.17
N$5
  Top 0.254: IC4.33 59.21,40.92 59.21,41.49 62.06,44.35 R7.2
N$6  (via drill 0.61)
  Top 0.61: IC4.44 49.26,42.63 47.89,42.63 46.18,44.35 L2.1 45.83,44.58 44.92,44.58 43.55,45.95 42.06,45.95 41.6,45.49 v41.6,39.66 | v54.18,35.2 56.01,35.2 57.61,33.6 59.09,33.6 IC4.24 | v43.43,20.23 43.43,21.37 41.6,23.2 v41.6,25.6
  Bottom 0.61: v54.18,35.2 51.55,32.58 51.55,26.98 44.81,20.23 v43.43,20.23 | v41.6,39.66 v41.6,25.6
N$7
  Top 0.254: R22.2 83.9,30.52 85.5,30.52 86.53,29.49 90.41,29.49 91.44,30.52 R20.1
N$8
  Top 0.813: J3.1 21.6,77.38 24.14,75.44 24.12,72.92 24.12,71.21 JP14.2
N$9  (via drill 0.61)
  Top 0.254: v49.95,35.04 49.95,37.49 48.23,39.2 47.55,39.2 IC4.3 | v49.95,27.55 49.38,27.55 45.95,24.12 45.83,24.12 45.61,23.89 45.61,21.26 47.21,19.66 47.21,18.06 52.92,12.34 73.5,12.34 74.41,13.26 74.41,17.72 80.7,24 93.61,24 96.58,26.98 v96.58,33.83 | v76.24,54.75 74.87,53.38 R3.1
  Bottom 0.254: v49.95,27.55 v49.95,35.04 | v96.58,33.83 96.58,34.18 90.3,40.46 90.3,51.44 90.64,51.78 90.64,53.72 88.81,55.55 77.04,55.55 v76.24,54.75
N$10  (via drill 0.61)
  Top 0.254: v43.66,42.29 43.89,42.29 44.46,41.72 44.46,40.46 45.49,39.43 45.72,39.43 46.63,38.52 47.43,38.52 IC4.4 | v46.98,49.38 v44.12,49.38 | v73.27,50.06 74.3,50.06 74.75,49.61 R4.1
  Bottom 0.254: v43.66,42.29 43.66,48.92 v44.12,49.38 | v46.98,49.38 48.46,50.86 49.84,50.86 53.72,46.98 71.32,46.98 71.55,46.75 72.24,46.75 73.27,47.78 v73.27,50.06
N$11  (via drill 0.61)
  Top 0.254: X1.2 96.47,75.32 R5.1 96.24,75.44 94.46,73.66 93.66,73.66 92.7,72.69 92.7,72.35 91.9,71.55 89.5,71.55 85.95,68.01 v85.95,66.06 | v83.33,63.44 83.33,59.55 82.64,58.86 82.53,58.86 80.92,57.26 80.92,56.24 78.07,53.38 77.72,53.38 R3.2
  Bottom 0.254: v85.95,66.06 v83.33,63.44
N$12  (via drill 0.61)
  Top 0.254: R6.1 93.95,75.32 93.95,76.24 92.81,77.38 92.81,78.64 93.95,79.78 X1.3 | v85.95,71.21 84.24,69.49 84.24,56.35 77.72,49.84 77.72,49.61 R4.2
  Bottom 0.254: v85.95,71.21 86.41,71.21 92.81,77.61 92.81,78.64 93.95,79.78 X1.3
N$13
  Top 0.254: IC4.6 47.43,36.92 45.38,36.92 44.35,37.95 43.2,37.95 C6.2
N$14
  Top 0.254: LED3.C 101.61,83.33 101.61,80.24 R18.2
N$15
  Top 0.254: C17.+ 70.64,56.58 70.64,58.41 69.27,59.78 69.27,60.35 IC1.2
N$16
  Top 0.254: IC1.6 74.3,59.44 75.89,57.84 77.15,57.84 78.41,56.58 79.1,56.58 C18.-
N$17
  Top 0.254: C15.- 65.04,56.58 65.72,56.58 66.75,57.61 68.69,57.61 69.49,56.81 69.49,55.66 69.72,55.44 71.67,55.44 71.89,55.66 71.89,58.41 70.52,59.78 70.52,60.35 IC1.3
N$18
  Top 0.254: C16.- 76.35,56.58 73.95,58.98 73.84,58.98 73.04,59.78 73.04,60.35 IC1.5
N$19
  Top 0.254: C16.+ 73.38,56.58 73.38,58.18 71.78,59.78 71.78,60.35 IC1.4
N$20
  Top 0.254: C15.+ 62.06,56.58 63.09,56.58 64.35,57.84 65.61,57.84 67.89,60.12 67.89,60.35 IC1.1
N$21
  Top 0.254: IC1.14 70.52,66.64 70.52,68.24 73.61,71.32 73.61,78.64 J1.4
N$22  (via drill 0.61)
  Top 0.254: v71.67,64.81 71.67,66.52 IC1.13 | v67.44,69.04 67.44,73.95 v70.18,76.69
  Bottom 0.254: v67.44,69.04 v71.67,64.81 | v70.18,76.69 71.32,76.69 71.89,77.27 73.84,77.27 74.87,76.24 J1.3
N$23
  Top 0.61: J1.2 76.24,78.64 77.5,78.64 81.27,74.87 81.27,71.21 JP2.2
N$24
  Top 0.254: J1.6 71.09,78.64 71.09,73.72 68.58,71.21 JP3.2
N$25
  Top 0.254: J1.1 77.5,76.12 77.5,71.21 JP4.2
N$26
  Top 0.813: J2.1 9.6,77.38 11.51,75.58 11.43,71.21 JP13.2
N$27
  Top 0.61: T1.3 71.67,4 69.61,4 64.81,8.8 SG1.-
N$28
  Top 0.254: R22.1 83.9,27.77 87.55,27.77 R21.2 87.67,27.89 88.81,29.03 92.01,29.03 92.7,29.72 92.7,32.35 97.16,36.8 98.98,36.8 JP18.1
N$29
  Top 0.254: OK1.1 11.43,65.84 10.97,65.84 8.34,68.47 R8.2
N$30
  Top 0.813: J4.1 33.72,77.38 36.26,75.51 36.12,71.21 JP19.2
N$31
  Top 0.813: J5.1 48.26,76.07 48.23,72.92 48.23,71.21 JP20.2
N$32
  Top 0.254: OK2.1 24.12,65.84 23.66,65.84 21.03,68.47 R9.2
N$33
  Top 0.813: U$1.P$2 96.58,66.06 97.04,66.06 105.39,74.41 F2.2 105.73,74.64 109.39,78.3 110.53,78.3 U$2.TIP
N$34
  Top 0.254: U$3.J1.1 92.7,46.98 98.98,46.98 JP16.2
N$35
  Top 0.254: OK3.1 35.55,65.84 33.03,68.35 R10.2
N$36
  Top 0.254: SV3.1 111.78,8.91 111.78,12.69 JP1.2
N$37
  Top 0.254: JP17.1 98.98,43.2 97.16,43.2 95.78,44.58 90.07,44.58 88.92,45.72 U$3.J1.2
N$38
  Top 0.254: OK4.1 48.23,65.84 47.78,65.84 45.15,68.47 R11.2
N$39
  Top 0.254: R27.1 91.44,61.15 95.21,61.15 R26.1 95.33,61.15 98.98,61.15 R25.2
N$40
  Top 0.254: T1.1 72.69,6.29 72.69,10.4 72.47,10.63 R19.1
N$41  (via drill 0.61)
  Top 0.254: v11.77,18.97 11.32,18.52 11.32,14.86 11.54,14.63 12.57,14.63 13.26,15.32 13.26,15.89 IC5.2 | v11.77,32.92 11.77,39.43 v11.32,39.89
  Bottom 0.254: 11.32,40.23 13.03,40.23 J6.CMD | 11.32,40.23 10.86,40.23 7.54,43.55 7.54,45.15 9.37,46.98 30.63,46.98 30.86,46.75 30.86,45.61 29.6,44.35 29.6,43.66 U1.2 | v11.77,32.92 v11.77,18.97 | 11.32,40.23 v11.32,39.89
N$42  (via drill 0.61)
  Top 0.254: v82.3,59.78 79.44,62.64 79.44,75.78 77.95,77.27 76.12,77.27 75.09,78.3 75.09,79.1 75.78,79.78 76.69,79.78 77.15,79.32 83.44,79.32 83.67,79.55 83.67,81.38 82.64,82.41 82.64,83.33 LED1.C | v92.58,42.06 87.1,36.58 68.69,36.58 66.29,34.18 66.29,31.77 R16.2
  Bottom 0.254: v82.3,59.78 83.44,59.78 87.21,56.01 89.04,56.01 92.58,52.46 v92.58,42.06
N$43
  Top 0.254: LED2.C 82.53,80.58 55.8,80.58 55.46,80.92 32.8,80.92 25.95,74.07 25.95,70.75 24.92,69.72 20,69.72 16.69,66.41 16.69,61.49 16.57,61.38 16.57,56.24 33.72,39.09 35.66,39.09 40.46,34.29 R17.2
N$44  (via drill 0.61)
  Top 0.254: v15.54,14.17 15.77,14.4 15.77,15.89 IC5.4 | v9.6,29.49 12.69,32.58 12.69,39.78 v11.32,41.15
  Bottom 0.254: 11.83,41.66 12.23,41.26 13.03,41.26 J6.DAT3 | 11.83,41.66 11.66,41.83 11.66,45.26 12.46,46.06 29.49,46.06 U1.1 | v15.54,14.17 14.06,14.17 9.6,18.63 v9.6,29.49 | 11.83,41.66 v11.32,41.15
N$45  (via drill 0.61)
  Top 0.254: v16.34,37.83 v17.95,36.23 17.95,36.12 v15.09,33.26 | v17.6,20.34 18.4,19.55 18.4,16 IC5.6
  Bottom 0.254: v17.95,36.23 29.49,36.23 U1.5 | v16.34,37.83 13.14,37.83 J6.CLK | v17.6,20.34 17.6,30.75 v15.09,33.26
N$46
  Top 0.254: D4.C 103.67,64.69 103.67,62.87 99.1,58.29 R25.1
N$47
  Top 0.254: Q3.1 87.33,53.26 87.33,58.18 Q2.1 87.44,58.18 91.44,58.18 R27.2
N$48
  Top 0.508: Q3.2 85.38,53.26 85.38,58.18 Q2.2
R2IN  (via drill 0.61)
  Top 0.254: v76.24,58.75 76.81,59.32 76.81,60.35 IC1.8 | v65.27,58.75 63.21,58.75 53.38,68.58 SV4.5
  Bottom 0.254: v65.27,58.75 v76.24,58.75
R2OUT  (via drill 0.61)
  Top 0.254: v67.09,62.75 73.61,62.75 76.81,65.95 76.81,66.52 IC1.9 | v62.87,64.01 62.87,64.24 58.52,68.58 SV4.3
  Bottom 0.254: v67.09,62.75 64.12,62.75 v62.87,64.01
RESET  (via drill 0.61)
  Top 0.254: IC4.13 50.06,30.98 50.06,30.18 49.84,29.95 45.38,29.95 45.15,30.18 D1.A 45.03,30.18 43.78,30.19 43.78,30.07 | v44.35,8.69 44.35,25.49 43.78,26.06 43.78,30.07 | 43.78,30.07 42.63,29.95 C3.1 42.52,30.06 40.12,30.06 C4.1 40.01,30.06 37.49,30.06 R2.1 37.38,29.95 36.23,28.8 36.23,25.26 35.2,24.23 v28.92,24.23 | v10.52,18.97 9.37,17.83 5.14,17.83 ISP1.5
  Bottom 0.254: v44.35,8.69 44.35,7.43 45.26,6.51 49.84,6.51 63.55,20.23 69.84,20.23 SV2.14 | v10.52,18.97 11.43,18.06 16.57,18.06 22.75,24.23 v28.92,24.23
RX_LED
  Top 0.254: IC4.8 47.43,35.2 44.35,35.2 43.43,34.29 R17.1
RXD1  (via drill 0.61)
  Top 0.254: JP4.1 74.87,71.09 73.04,69.27 73.04,66.64 IC1.12 73.04,66.52 v73.04,64.81 | v63.42,24.11 61.96,24.11 55.78,30.29 55.78,30.98 IC4.20 | v75.32,17.26 75.32,7.43 80.24,2.52 102.41,2.52 108.7,8.8 109.16,8.8 SV3.2 | v106.19,50.63 112.58,44.23 v112.58,39.89
  Bottom 0.254: v63.42,24.11 67.32,24.11 69.84,22.86 SV2.13 69.84,22.75 v75.32,17.26 | v73.04,64.81 80.7,64.81 87.9,57.61 99.21,57.61 v106.19,50.63 | v112.58,39.89 112.58,14.06 112.81,13.83 112.81,11.54 111.9,10.63 110.98,10.63 109.27,8.91 SV3.2
SCK  (via drill 0.61)
  Top 0.254: IC4.9 47.43,34.4 45.72,34.4 44.35,33.03 36.8,33.03 34.29,35.55 SV1.8 34.18,35.55 18.63,35.55 1.37,18.29 1.37,17.26 1.42,16.57 1.42,16.46 | v19.77,12.34 19.77,15.89 IC5.7 | 1.42,16.46 1.37,15.77 1.37,14.74 1.42,14.06 3.49,14.06 3.77,13.78 3.77,12.34 5.94,10.17 12.69,10.17 X2.2 | 1.42,16.46 3.89,16.46 5.03,15.32 ISP1.3
  Bottom 0.254: v19.77,12.34 21.49,10.63 21.49,7.2 20.57,6.29 14.52,6.29 13.6,5.37 11.66,5.37 6.29,10.74 6.29,14.06 5.14,15.2 ISP1.3
SCL  (via drill 0.61)
  Top 0.254: U$3.J2.1 88.81,10.06 88.81,6.29 86.41,3.89 I2C_DISPLEJ.SCL | v54.34,28.22 54.18,28.38 54.18,30.98 IC4.18 | v78.3,28.8 80.01,30.52 R23.2 | v81.15,32.12 81.15,31.89 80.01,30.75 R23.2 | v91.44,24.92 82.98,24.92 81.27,26.63 81.27,28.92 79.9,30.29 R23.2
  Bottom 0.254: v54.34,28.22 56.45,28.22 59.89,31.66 68.35,31.66 69.49,30.52 69.84,30.52 SV2.10 69.72,30.4 68.12,28.8 68.12,27.55 68.81,26.86 70.87,26.86 72.81,28.8 v78.3,28.8 | v81.15,32.12 83.33,34.29 83.33,36.01 86.3,38.98 86.3,45.72 U$3.J1.3 | v91.44,24.92 88.92,22.4 88.92,10.17 U$3.J2.1
SDA  (via drill 0.61)
  Top 0.254: v55.14,32.58 54.98,31.77 54.98,31.09 IC4.19 | v72.47,30.63 76.12,30.63 R24.2 | v86.3,23.09 v86.3,18.06
  Bottom 0.254: I2C_DISPLEJ.SDA 88.81,3.89 86.41,6.29 86.41,10.06 U$3.J2.2 86.3,10.17 v86.3,18.06 | v55.14,32.58 68.12,32.58 69.15,31.55 70.87,31.55 71.55,30.86 71.55,30.63 | 71.55,30.63 71.55,29.6 69.95,28 SV2.11 | 71.55,30.63 v72.47,30.63 80.92,30.63 | U$3.J1.4 84.81,45.72 85.95,46.86 86.75,46.86 87.55,46.06 87.55,39.55 83.78,35.78 83.78,33.49 80.92,30.63 | v86.3,23.09 86.3,25.15 80.92,30.52 80.92,30.63
T2IN
  Top 0.254: IC1.10 75.55,66.52 75.55,65.95 73.27,63.66 64.47,63.66 61.04,67.09 61.04,68.58 SV4.2
T2OUT
  Top 0.254: IC1.7 75.55,60.47 75.55,61.04 74.75,61.84 67.32,61.84 65.15,59.66 64.47,59.66 55.89,68.24 55.89,68.58 SV4.4
TX_LED
  Top 0.254: IC4.22 57.38,30.98 58.12,30.98 59.26,29.83 61.49,29.83 63.32,31.66 R16.1
TXD1  (via drill 0.61)
  Top 0.254: IC1.11 74.3,67.67 v76.24,69.61 76.35,69.61 v78.52,67.44 | v64.12,29.38 57.49,29.38 56.58,30.29 56.58,30.98 IC4.21 | v66.18,29.38 66.18,29.15 69.84,25.49 SV2.12 | v83.78,11.66 89.38,11.66 94.75,6.29 104.81,6.29 106.64,8.12 106.64,8.8 SV3.3 | v76.69,18.75 v81.38,14.06 | v110.87,43.55 110.87,42.29 111.56,41.6 111.56,38.85 v111.33,38.62
  Bottom 0.254: v76.24,69.61 75.67,69.61 75.32,69.27 73.04,69.27 71.21,71.09 JP3.1 | v66.18,29.38 v64.12,29.38 | v81.38,14.06 v83.78,11.66 | v76.69,18.75 69.95,25.49 SV2.12 | v78.52,67.44 85.84,67.44 95.21,58.06 106.3,58.06 110.87,53.49 v110.87,43.55 | v111.33,38.62 111.33,14.52 110.3,13.49 110.3,11.54 109.39,10.63 108.47,10.63 106.76,8.91 SV3.3
U-NAP
  Top 0.813: D4.A 107.1,64.81 107.1,66.18 105.5,67.78 F2.1 105.84,68.01 109.5,71.67 D2.A
VBUS  (via drill 0.61)
  Top 0.508: D3.C 85.15,77.04 85.15,75.44 86.87,73.72 F1.2 86.98,73.5 86.98,69.95 84.92,67.89 84.92,63.99 89.37,59.55 92.58,59.55 92.81,59.32 92.81,57.26 92.19,56.64 89.66,56.64 v88.7,54.41 | v86.41,54.63 86.41,56.01 Q2.3 | v89.72,52.12 91.33,52.12 91.44,52.01 C5.2 91.67,52.12 94.07,52.12 96.36,54.41 C7.+ 96.58,54.52 101.04,50.06 v101.04,44.91 | v44.92,36.12 47.43,36.12 IC4.7 | v40.58,23.2 40.58,15.09 41.95,13.72 41.95,5.71 v41.49,5.26 | v88.01,19.09 88.35,19.09 92.58,23.32 93.84,23.32 98.98,28.46 v98.98,31.77
  Bottom 0.508: v86.41,54.63 88.12,54.63 88.53,54.23 | 88.53,54.23 89.72,53.03 v89.72,52.12 | v88.7,54.41 88.53,54.23 | v44.92,36.12 44.92,27.55 v40.58,23.2 | v41.49,5.26 41.83,5.26 42.06,5.03 70.98,5.03 85.04,19.09 v88.01,19.09 | v98.98,31.77 101.04,33.83 v101.04,44.91
VIN
  Top 0.813: D2.C 113.96,71.67 113.04,71.67 108.7,67.32 108.7,62.87 107.1,61.27 C8.2 106.87,60.92 106.87,60.12 112.36,54.63 C12.+ 111.67,54.75 108.7,51.78 105.73,51.78 105.04,51.09 105.04,49.95 108.93,46.06 DC1.1 109.16,45.72 104.47,41.03 104.47,32.8 IC3.1
  Bottom 0.813: SV4.1 66.29,68.58 73.95,60.92 83.44,60.92 87.55,56.81 98.41,56.81 105.73,49.49 106.64,49.49 107.33,50.18 107.33,53.61 108.01,54.29 108.93,54.29 109.61,53.61 109.61,46.06 109.27,45.72 DC1.1
(copper drawn outside any net)
  shapes: Top area x4

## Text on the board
Bottom: B-0090 | v1.0 | Stopky v4.1 | www.sakul.cz
tPlace: 12V | 12V | 12V | 12V | VIN | R2IN | T2OUT | R2OUT | T2IN | TL.1 | TL.2 | TL.3 | A0 | IN1 | IN2 | A1 | IN3 | A2 | A3 | IN4 | A4 | D13 | A5 | 1 | D12 | v1.0 | CS | D7 | SCK | D6 | MOSI | D5 | SCL | MISO | 2xGND | SDA | TXD1 | Stopky v4.1 | B-0090 | www.sakul.cz | 2x5V | RXD1 | RES. | R | 3V3 | AREF | GND | MO | SCK | 5V | MI | 5V | GND | RX | TX | SET | SD KARTA | LED DISPLEJ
